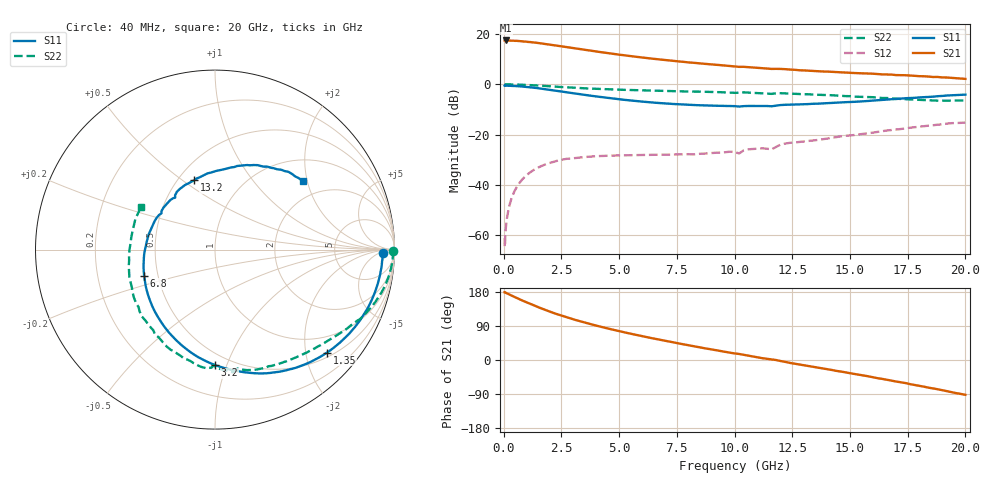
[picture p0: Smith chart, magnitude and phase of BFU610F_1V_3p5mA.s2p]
! Filename:  P:\Prog\Test\Noise\ATS_data\Testdata_Net\SplitFiles\BFU610_2W_A5_HighFreq_1V_3.5mA_D.s2p
! Date/Time: Wed 10/Aug/2011 16:54:40
! BFU610_2W_A5_HighFreq_1V_1mA_10mA_Bias3_R.s2p
! MDIF S-parameter v. bias file
! BFU610_2W_A5_HighFreq_1V_1mA_10mA
! Date/time Mon Aug 08 13:53:02 2011
! VAR V_out= 1.0001
! VAR I_out= 3.4950
! VAR V_in= 0.8933
! VAR I_in= 0.0280
! Device data file deembeded for feedlines and parallel
! Original file: \SplitFiles\BFU610_2W_A5_HighFreq_1V_3.5mA_R.s2p
! Feed-files: PR003V01_101208_Feed1.s2p, PR003V01_101208_Feed2.s2p
! Parallel-file: PR003V01_101208_Par.s2p
# MHz S MA R 50
!  Freq-MHz  S11-mag  S11-arg  S21-mag  S21-arg  S12-mag  S12-arg  S22-mag  S22-arg
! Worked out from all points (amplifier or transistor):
!   167 points, 40 MHz to 20 GHz, reference 50 ohm
!   highest |S21| = 17.3 dB at 80 MHz (marker M1)
!   |S21| within 3 dB of that: start of sweep to 2.979 GHz
!   unconditionally stable (mu >= 1): 4.922 GHz to end of sweep
!   at 550 MHz: K = 0.06, MSG = 29.1 dB, |S12| = -41.0 dB
!   at 4.2 GHz: K = 0.83, MSG = 20.6 dB, |S12| = -28.5 dB
!   at 20 GHz: K = 1.05, MAG = 7.3 dB, |S12| = -15.2 dB
!   S11 on the Smith chart (normalised r, x): 40 MHz: 26, -9; 1.35 GHz: 0.60, -2.44; 3.2 GHz: 0.41, -0.91; 6.8 GHz: 0.42, -0.15; 13.2 GHz: 0.60, +0.55; 20 GHz: 1.50, +1.87
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40  0.9343 -1.3  7.365 179.0  0.000613 87.3  0.9905 -0.4
60  0.9346 -1.7  7.357 178.0  0.0006924 87.6  0.9916 -0.6
80  0.9335 -2.6  7.37 177.7  0.001192 90.3  0.9918 -0.9
220  0.9312 -7.2  7.339 173.6  0.003454 88.2  0.991 -2.8
440  0.9228 -14.4  7.27 167.3  0.0071 83.9  0.987 -5.6
950  0.8863 -30.6  7.003 153.2  0.01507 72.7  0.9687 -11.9
1350  0.8476 -42.6  6.697 143.0  0.02049 64.8  0.948 -16.4
1750  0.8038 -53.9  6.341 133.3  0.02505 57.9  0.9251 -20.6
2150  0.758 -64.7  5.968 124.4  0.02862 51.9  0.9025 -24.6
2700  0.6936 -78.4  5.47 113.3  0.03297 43.9  0.8667 -29.2
3200  0.6438 -89.9  5.032 104.1  0.03471 38.8  0.8424 -33.1
3400  0.6248 -94.3  4.881 100.7  0.0355 37.1  0.8336 -34.6
4100  0.5646 -109.2  4.393 89.3  0.03751 31.9  0.8062 -39.4
4900  0.5085 -124.8  3.913 77.6  0.0386 27.9  0.7819 -44.8
5800  0.4602 -141.8  3.471 65.4  0.03934 25.0  0.7593 -50.7
6800  0.4209 -159.6  3.077 53.0  0.03983 23.9  0.7387 -57.3
8600  0.3805 170.4  2.567 32.3  0.0418 26.6  0.7097 -69.4
10200  0.3603 145.9  2.207 15.9  0.04237 31.2  0.6765 -79.4
13200  0.4032 106.9  1.854 -15.8  0.07441 30.4  0.6314 -105.7
13400  0.4091 104.7  1.827 -17.8  0.07655 29.8  0.6219 -108.0
16800  0.5038 69.2  1.551 -54.5  0.1233 12.7  0.5249 -149.3
20000  0.6209 38.2  1.275 -92.0  0.1737 -17.6  0.4751 150.1
